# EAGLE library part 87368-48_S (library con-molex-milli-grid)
RECEPTACAL
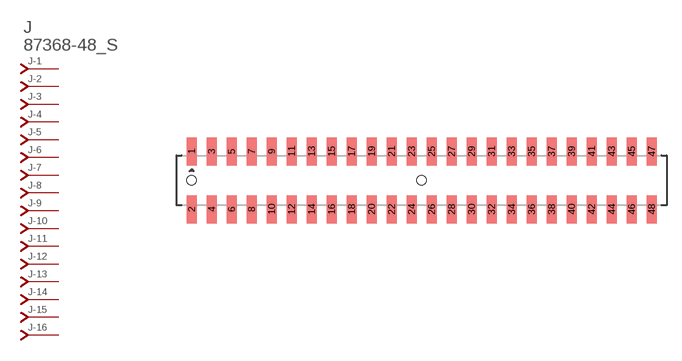
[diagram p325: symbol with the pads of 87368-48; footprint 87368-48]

Designator prefix J; gates -1=J-NV -2=J-N -3=J-N -4=J-N -5=J-N -6=J-N -7=J-N -8=J-N -9=J-N -10=J-N -11=J-N -12=J-N -13=J-N -14=J-N -15=J-N -16=J-N -17=J-N -18=J-N -19=J-N -20=J-N -21=J-N -22=J-N -23=J-N -24=J-N -25=J-N -26=J-N -27=J-N -28=J-N -29=J-N -30=J-N -31=J-N -32=J-N -33=J-N -34=J-N -35=J-N -36=J-N -37=J-N -38=J-N -39=J-N -40=J-N -41=J-N -42=J-N -43=J-N -44=J-N -45=J-N -46=J-N -47=J-N -48=J-N

## 87368-48_S  [87368-48]
1  -1:J  pas
2  -2:J  pas
3  -3:J  pas
4  -4:J  pas
5  -5:J  pas
6  -6:J  pas
7  -7:J  pas
8  -8:J  pas
9  -9:J  pas
10  -10:J  pas
11  -11:J  pas
12  -12:J  pas
13  -13:J  pas
14  -14:J  pas
15  -15:J  pas
16  -16:J  pas
17  -17:J  pas
18  -18:J  pas
19  -19:J  pas
20  -20:J  pas
21  -21:J  pas
22  -22:J  pas
23  -23:J  pas
24  -24:J  pas
25  -25:J  pas
26  -26:J  pas
27  -27:J  pas
28  -28:J  pas
29  -29:J  pas
30  -30:J  pas
31  -31:J  pas
32  -32:J  pas
33  -33:J  pas
34  -34:J  pas
35  -35:J  pas
36  -36:J  pas
37  -37:J  pas
38  -38:J  pas
39  -39:J  pas
40  -40:J  pas
41  -41:J  pas
42  -42:J  pas
43  -43:J  pas
44  -44:J  pas
45  -45:J  pas
46  -46:J  pas
47  -47:J  pas
48  -48:J  pas

## Footprint 87368-48 (pad centres in mm)
RECEPTACAL SMD Dual Row, Side Entry
smd 1 x 2.8: 1 -23,2.9; 2 -23,-2.9; 3 -21,2.9; 4 -21,-2.9; 5 -19,2.9; 6 -19,-2.9; 7 -17,2.9; 8 -17,-2.9; 9 -15,2.9; 10 -15,-2.9; 11 -13,2.9; 12 -13,-2.9; 13 -11,2.9; 14 -11,-2.9; 15 -9,2.9; 16 -9,-2.9; 17 -7,2.9; 18 -7,-2.9; 19 -5,2.9; 20 -5,-2.9; 21 -3,2.9; 22 -3,-2.9; 23 -1,2.9; 24 -1,-2.9; 25 1,2.9; 26 1,-2.9; 27 3,2.9; 28 3,-2.9; 29 5,2.9; 30 5,-2.9; 31 7,2.9; 32 7,-2.9; 33 9,2.9; 34 9,-2.9; 35 11,2.9; 36 11,-2.9; 37 13,2.9; 38 13,-2.9; 39 15,2.9; 40 15,-2.9; 41 17,2.9; 42 17,-2.9; 43 19,2.9; 44 19,-2.9; 45 21,2.9; 46 21,-2.9; 47 23,2.9; 48 23,-2.9
hole 0.914 at -23,0
hole 0.914 at 0,0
